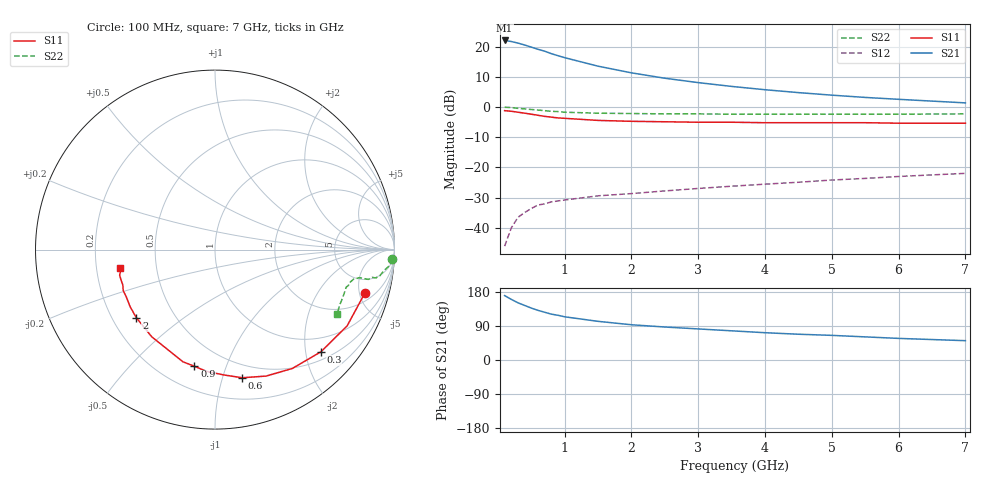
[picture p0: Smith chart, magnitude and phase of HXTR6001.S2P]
! HXTR-6001 Common Emitter
! Vce=10V Ic=4mA
# ghz s ma r 50
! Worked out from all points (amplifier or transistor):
!   21 points, 100 MHz to 7 GHz, reference 50 ohm
!   highest |S21| = 22.0 dB at 100 MHz (marker M1)
!   |S21| within 3 dB of that: start of sweep to 612.3 MHz
!   unconditionally stable (mu >= 1): 2.487 GHz to end of sweep
!   at 400 MHz: K = 0.19, MSG = 27.7 dB, |S12| = -34.9 dB
!   at 1.5 GHz: K = 0.71, MSG = 21.4 dB, |S12| = -29.4 dB
!   at 7 GHz: K = 1.35, MAG = 8.1 dB, |S12| = -21.9 dB
!   S11 on the Smith chart (normalised r, x): 100 MHz: 2.88, -5.69; 300 MHz: 0.66, -2.31; 600 MHz: 0.38, -1.16; 900 MHz: 0.34, -0.78; 2 GHz: 0.30, -0.34; 7 GHz: 0.30, -0.09
0.1  0.87 -16.0  12.6 170.0  0.005 82.0  0.99 -3.0
0.2  0.85 -30.0  12.1 160.0  0.01 75.0  0.98 -5.0
0.3  0.82 -44.0  11.4 151.0  0.015 68.0  0.95 -7.0
0.4  0.79 -57.0  10.6 144.0  0.018 63.0  0.93 -9.0
0.5  0.76 -68.0  9.77 137.0  0.021 58.0  0.91 -10.0
0.6  0.73 -78.0  9 131.0  0.024 55.0  0.89 -10.0
0.7  0.7 -86.0  8.37 126.0  0.025 52.0  0.87 -11.0
0.8  0.68 -94.0  7.62 121.0  0.027 50.0  0.85 -11.0
0.9  0.66 -100.0  7.05 118.0  0.028 48.0  0.84 -11.0
1  0.65 -106.0  6.54 114.0  0.029 47.0  0.82 -11.0
1.5  0.6 -126.0  4.73 102.0  0.034 45.0  0.79 -12.0
2  0.58 -139.0  3.67 93.0  0.037 45.0  0.78 -13.0
2.5  0.57 -146.0  2.99 87.0  0.041 47.0  0.77 -14.0
3  0.56 -152.0  2.53 82.0  0.045 49.0  0.77 -15.0
3.5  0.56 -156.0  2.19 77.0  0.049 51.0  0.76 -16.0
4  0.55 -159.0  1.93 72.0  0.053 52.0  0.76 -18.0
4.5  0.55 -162.0  1.73 68.0  0.057 53.0  0.76 -19.0
5  0.55 -164.0  1.57 65.0  0.062 54.0  0.76 -21.0
5.5  0.55 -165.0  1.44 61.0  0.066 55.0  0.76 -23.0
6  0.54 -167.0  1.34 57.0  0.071 55.0  0.76 -24.0
7  0.54 -169.0  1.17 51.0  0.08 56.0  0.77 -28.0
